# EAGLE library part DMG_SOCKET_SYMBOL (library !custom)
Super lazy 1-time-use symbol for the all-in-one schematic of the DMG
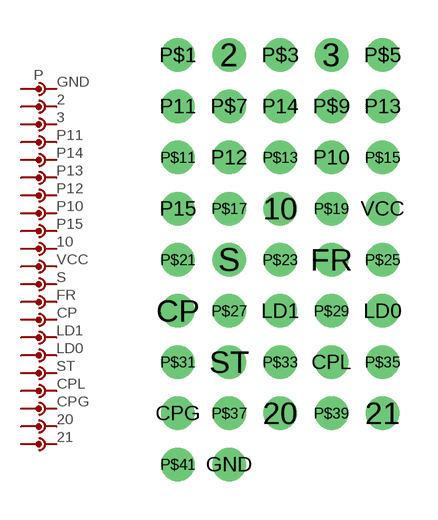
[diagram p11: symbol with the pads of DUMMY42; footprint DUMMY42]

Designator prefix P

## DMG_SOCKET_SYMBOL  [DUMMY42]
2  2  pas
3  3  pas
10  10  pas
20  20  pas
21  21  pas
CP  14  pas
CPG  19  pas
CPL  18  pas
FR  13  pas
GND  GND  pas
LD0  16  pas
LD1  15  pas
P10  8  pas
P11  4  pas
P12  7  pas
P13  6  pas
P14  5  pas
P15  9  pas
P$1  2  pas
P$3  3  pas
P$5  4  pas
P$7  5  pas
P$9  6  pas
P$11  7  pas
P$13  8  pas
P$15  9  pas
P$17  10  pas
P$19  11  pas
P$21  12  pas
P$23  13  pas
P$25  14  pas
P$27  15  pas
P$29  16  pas
P$31  17  pas
P$33  18  pas
P$35  19  pas
P$37  20  pas
P$39  21  pas
P$41  GND  pas
S  12  pas
ST  17  pas
VCC  11  pas

## Footprint DUMMY42 (pad centres in mm)
drill 0.8: 2 2,0; 3 6,0; 10 4,-6; 20 4,-14; 21 8,-14; CP 0,-10; CPG 0,-14; CPL 6,-12; FR 6,-8; GND 2,-16; LD0 8,-10; LD1 4,-10; P10 6,-4; P11 0,-2; P12 2,-4; P13 8,-2; P14 4,-2; P15 0,-6; P$1 0,0; P$3 4,0; P$5 8,0; P$7 2,-2; P$9 6,-2; P$11 0,-4; P$13 4,-4; P$15 8,-4; P$17 2,-6; P$19 6,-6; P$21 0,-8; P$23 4,-8; P$25 8,-8; P$27 2,-10; P$29 6,-10; P$31 0,-12; P$33 4,-12; P$35 8,-12; P$37 2,-14; P$39 6,-14; P$41 0,-16; S 2,-8; ST 2,-12; VCC 8,-6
